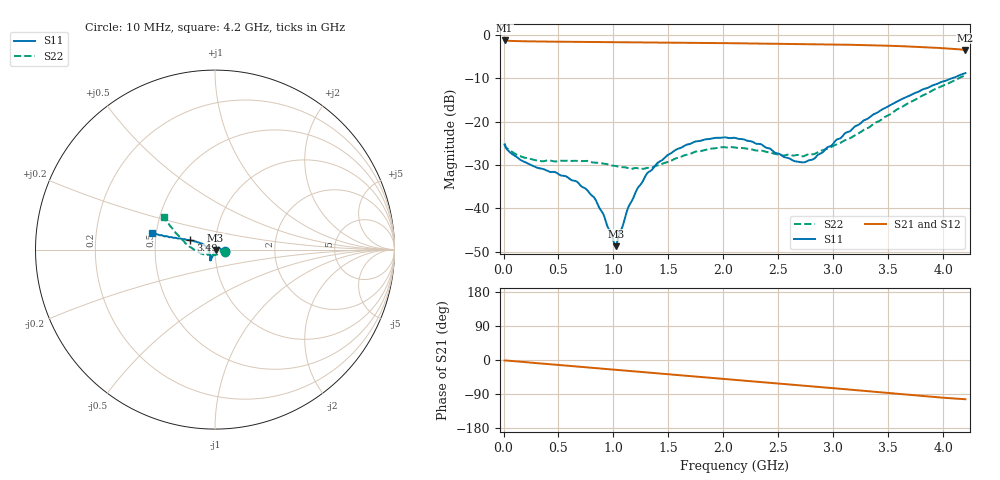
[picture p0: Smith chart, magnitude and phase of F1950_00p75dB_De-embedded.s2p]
! Integrated Device Technology
! Corporate Headquarters
! 6024 Silver Creek Valley Road
! San Jose, CA 95138  USA
! Phone:  1-408-284-8200
! Toll Free:  1-800-223-1366
! Webpage:  http://www.idt.com/
! Timing and RF Division
! 515 Groton Road, Suite 102
! Westford, MA 01886-6024
! Device:  F1950
! Description: 7-bit 0.25 dB Digital Step Attenuator
! Frequency:  150.0 -  4000.00 MHz
! Package:  4x4 mm Thin QFN Plastic Package: 24 pin
! Ports:  2 RF, 12 DC
!  Pin  1  = D0
!  Pin  2  = VDD
!  Pin  3  = Vmode
!  Pin  4  = GND
!  Pin  5  = RF1  =  Port 1
!  Pin  6  = GND
!  Pin  7  = GND
!  Pin  8  = GND
!  Pin  9  = GND
!  Pin 10  = GND
!  Pin 11  = GND
!  Pin 12  = GND
!  Pin 13  = GND
!  Pin 14  = RF2  =  Port 2
!  Pin 15  = GND
!  Pin 16  = LE
!  Pin 17  = CLK
!  Pin 18  = DATE
!  Pin 19  = D6
!  Pin 20  = D5
!  Pin 21  = D4
!  Pin 22  = D3
!  Pin 23  = D2
!  Pin 24  = D1
! State:  3
! Atten State:  0.75 dB
! Voltage:  +5.00 Volts
! Current:  Not Measured mA
! Data:  The device was measured on a the F195X evaluation board which has
!  individual transmission lines to the RF pins.  Data was collected
!  using a calibrated network analyzer.  The evaluation board was
!  de-embedded using a TRL calibration technique.
!  The reference plane is the edge of the package pin.
! Misc:  Board 2019
!  Action Tracker AT0250
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# GHz S dB R 50
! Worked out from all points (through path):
!   420 points, 10 MHz to 4.2 GHz, reference 50 ohm
!   highest |S21| = -1.35 dB at 10 MHz (marker M1); lowest = -3.5 dB at 4.2 GHz (marker M2)
!   group delay of S21, straight-line fit = 68.6 ps
!   lowest |S11| = -48.7 dB at 1.02 GHz (marker M3), VSWR 1.01, Z = 50.3 - j0.2 ohm
!   |S11| at or under -10 dB: start of sweep to 4.083 GHz
!   |S22| runs from -30.9 to -9.4 dB; largest |S21 - S12| = 0.001
!   S11 on the Smith chart (normalised r, x): 10 MHz: 1.11, -0.02; 3.49 GHz: 0.75, +0.08; 4.2 GHz: 0.48, +0.10
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0.01  -25.31 -11.3  -1.35 -1.2  -1.35 -1.2  -25.07 -11.7
0.12  -28.16 -7.7  -1.50 -3.7  -1.50 -3.7  -27.63 -7.5
0.29  -30.48 8.9  -1.58 -7.9  -1.58 -8.0  -28.93 -3.6
0.57  -32.63 31.6  -1.65 -14.7  -1.65 -14.7  -29.02 -1.2
0.71  -34.96 37.0  -1.68 -18.1  -1.67 -18.1  -29.11 -8.2
0.83  -37.69 36.4  -1.70 -21.0  -1.70 -21.0  -29.46 -15.4
1.02  -48.69 -32.6  -1.73 -25.6  -1.73 -25.7  -30.23 -35.3
1.04  -47.04 -55.3  -1.74 -26.1  -1.74 -26.1  -30.38 -38.4
1.13  -40.02 -95.2  -1.76 -28.3  -1.75 -28.3  -30.70 -51.2
1.21  -35.78 -104.8  -1.77 -30.2  -1.77 -30.2  -30.71 -64.4
1.3  -32.13 -108.5  -1.79 -32.4  -1.79 -32.4  -30.72 -80.3
1.41  -29.36 -109.9  -1.81 -35.1  -1.81 -35.1  -30.05 -98.2
1.57  -26.46 -111.4  -1.85 -39.0  -1.85 -39.0  -28.46 -119.1
1.74  -24.64 -112.3  -1.89 -43.2  -1.89 -43.2  -26.97 -134.1
2.11  -23.80 -114.7  -1.99 -52.2  -1.99 -52.3  -26.01 -150.2
2.34  -25.22 -121.0  -2.06 -57.8  -2.06 -57.9  -26.68 -151.2
2.66  -29.20 -153.1  -2.14 -65.7  -2.14 -65.8  -27.73 -142.8
2.81  -28.76 -179.2  -2.20 -69.5  -2.19 -69.5  -27.55 -140.9
3.15  -22.25 156.5  -2.34 -78.2  -2.34 -78.3  -23.87 -155.2
3.49  -16.63 159.4  -2.56 -87.0  -2.55 -87.1  -18.68 -179.6
3.51  -16.34 159.7  -2.57 -87.5  -2.57 -87.6  -18.43 179.2
4.2  -8.85 165.2  -3.51 -103.5  -3.50 -103.6  -9.39 147.4
